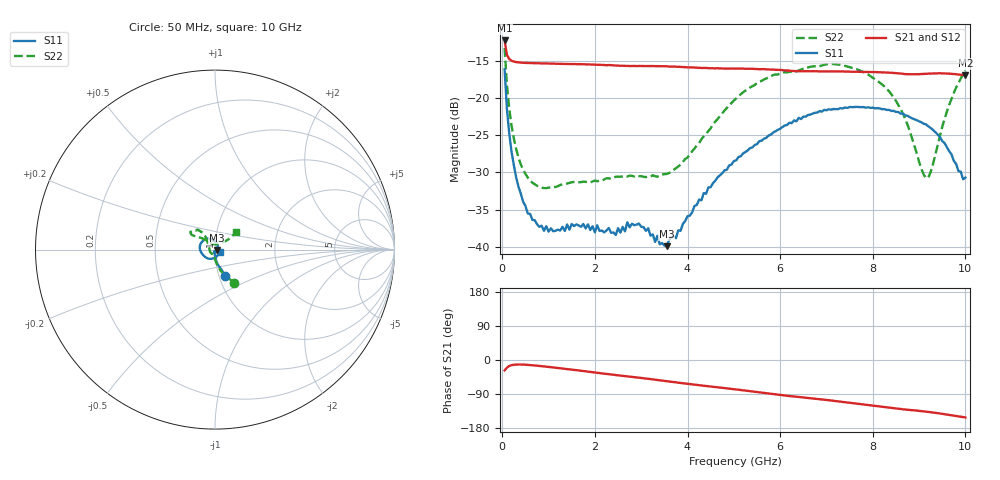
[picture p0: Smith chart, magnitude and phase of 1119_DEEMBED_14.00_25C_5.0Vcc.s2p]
!Hittite Microwave Corp.
!Digital Attenuator/PhaseShifter Rev 1.4.0
!Filename: C:\DATA\DATA\1119_DEEMBED_14.00_25C_5.0Vcc.s2p
!VNA ID: Agilent Technologies,N5224A,MY51441122,A.10.45.03
!Device type:
!2 Port Calibration.
!Temp(C): 25
!Lot Number:
!Serial Number:
!Operator:
!Misc:
!Attenuator:  14.000
# GHZ S DB R 50.0
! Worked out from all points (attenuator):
!   200 points, 50 MHz to 10 GHz, reference 50 ohm
!   highest |S21| = -12.30 dB at 50 MHz (marker M1); lowest = -17.0 dB at 10 GHz (marker M2)
!   lowest |S11| = -39.9 dB at 3.55 GHz (marker M3), VSWR 1.02, Z = 51 - j0.244 ohm
!   |S11| at or under -10 dB: start of sweep to end of sweep
!   |S22| runs from -32.1 to -13.3 dB; largest |S21 - S12| = 0.00043
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0.05  -16.15 -68.1  -12.30 -27.5  -12.30 -27.5  -13.33 -60.3
0.1  -21.50 -79.7  -14.23 -20.2  -14.23 -20.2  -18.23 -75.2
0.2  -27.23 -88.0  -15.02 -13.7  -15.02 -13.7  -23.74 -86.6
0.35  -31.92 -93.3  -15.24 -11.8  -15.24 -11.8  -28.02 -93.5
0.55  -35.49 -100.2  -15.32 -12.8  -15.32 -12.8  -30.67 -99.6
0.9  -37.82 -106.0  -15.38 -16.9  -15.38 -16.9  -32.09 -105.8
1.75  -36.91 -111.5  -15.49 -29.1  -15.49 -29.1  -31.23 -115.6
2.45  -38.38 -91.5  -15.66 -39.7  -15.67 -39.8  -30.57 -134.2
2.95  -36.84 -73.5  -15.72 -46.6  -15.73 -46.7  -30.48 -152.8
3.4  -39.64 -40.5  -15.75 -53.5  -15.76 -53.6  -30.42 -175.5
3.55  -39.88 -13.7  -15.76 -56.0  -15.77 -56.1  -30.19 175.9
4.35  -32.76 44.2  -15.98 -67.7  -16.00 -67.8  -25.17 136.4
5.05  -28.38 77.4  -16.07 -77.7  -16.09 -77.8  -20.07 126.1
5.85  -24.64 108.5  -16.21 -90.0  -16.22 -90.1  -16.93 130.3
6.7  -22.12 132.7  -16.42 -101.4  -16.44 -101.4  -15.78 139.8
7.65  -21.20 162.1  -16.50 -115.0  -16.51 -115.1  -16.14 147.6
8.35  -21.61 -178.9  -16.62 -125.7  -16.63 -125.7  -19.11 141.8
8.65  -22.10 -167.5  -16.77 -130.2  -16.76 -130.2  -22.10 135.3
9.1  -23.47 -139.7  -16.78 -135.5  -16.80 -135.5  -30.29 103.0
9.2  -23.82 -131.7  -16.75 -137.0  -16.77 -137.0  -30.67 81.0
9.65  -27.15 -88.0  -16.75 -144.9  -16.77 -144.9  -20.95 37.5
10  -30.69 -24.9  -16.97 -151.6  -16.98 -151.6  -16.34 39.5
